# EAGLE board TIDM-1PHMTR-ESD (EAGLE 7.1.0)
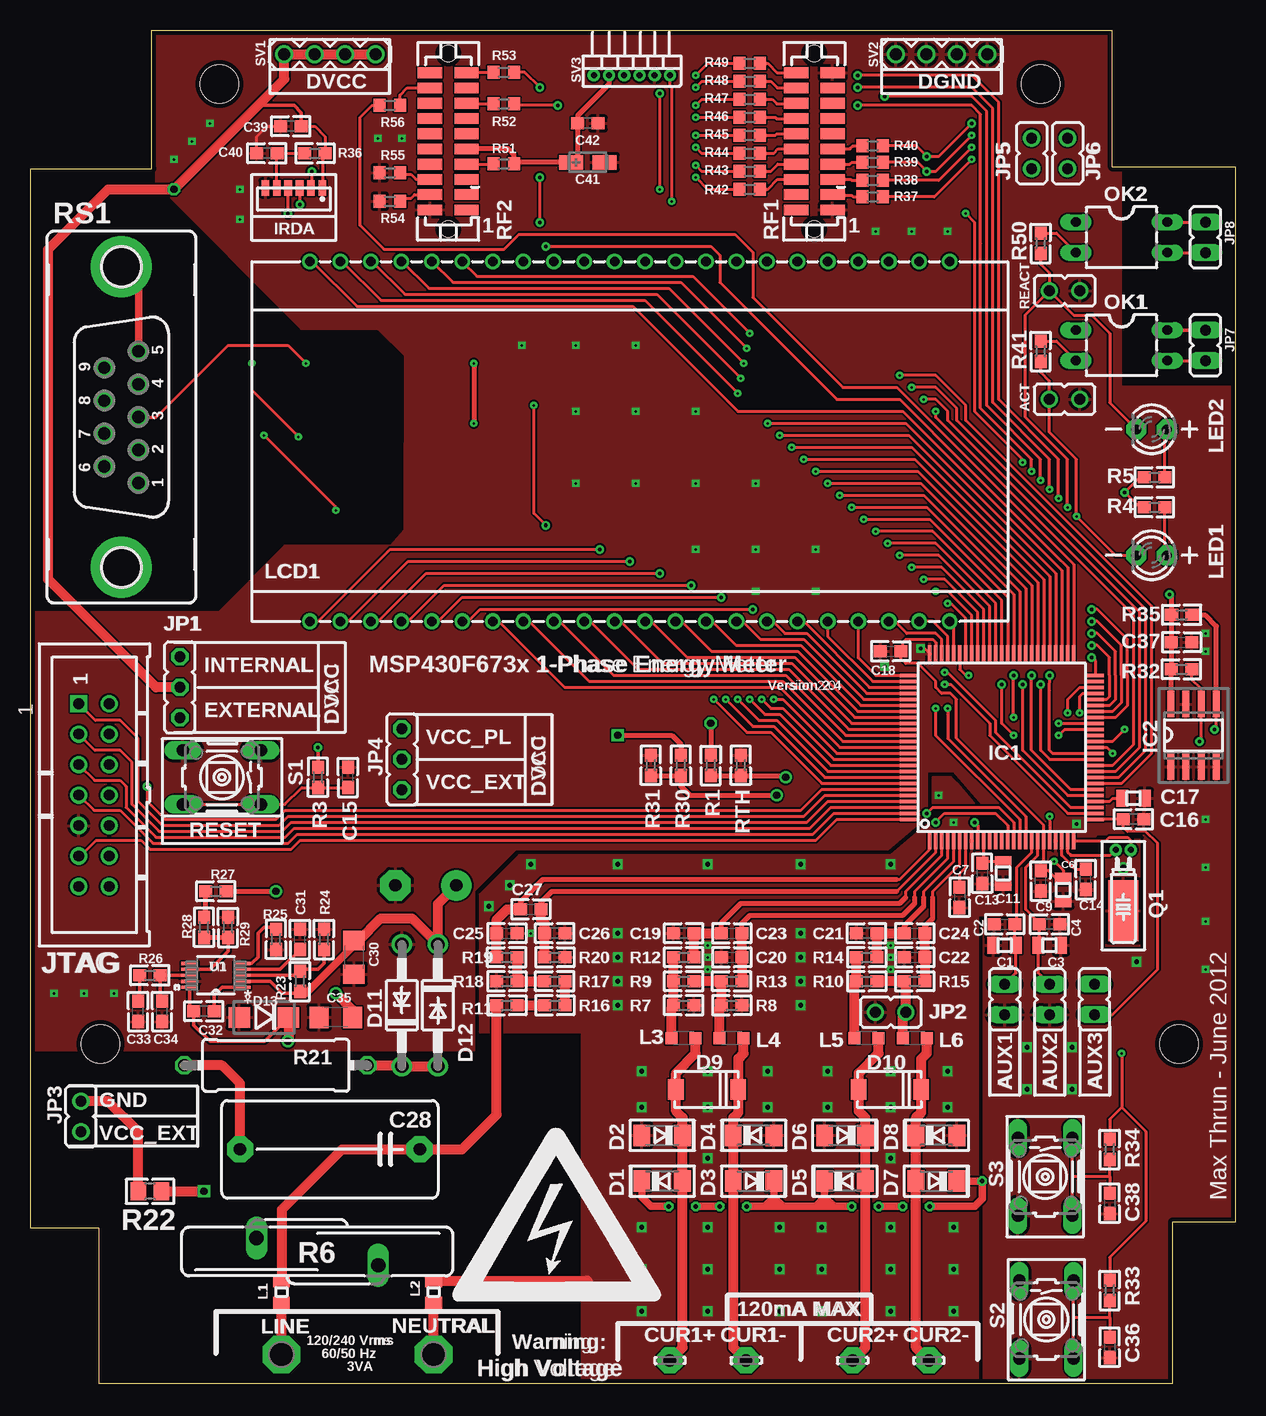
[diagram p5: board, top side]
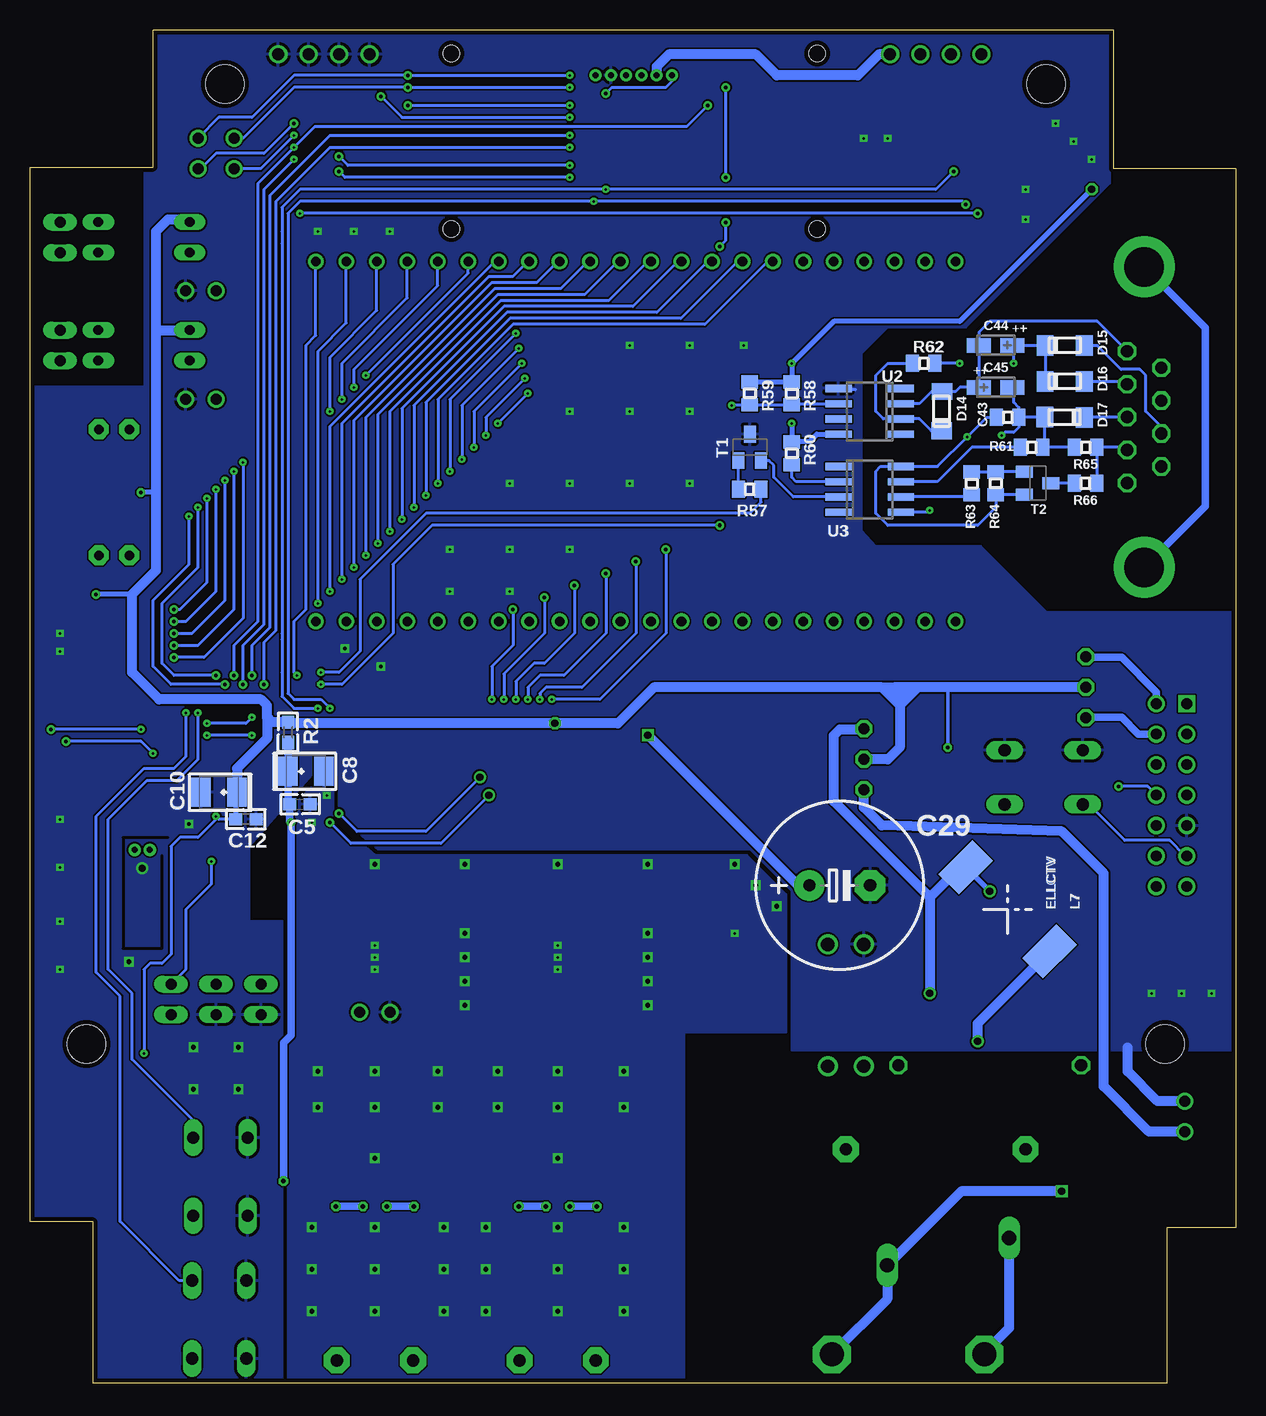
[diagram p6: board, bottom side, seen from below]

Size 100.51 x 112.78 mm. Coordinates in mm from the lower left corner, seen from the top.
Outline: 95.25,0 95.25,13.46 100.51,13.46 100.51,101.35 90.25,101.35 90.25,112.78 10.16,112.78 10.16,101.22 0,101.22 0,12.95 5.74,12.95 5.74,0 95.25,0
Copper layers (1*16): Top 0.0356mm / dielectric 1.5011mm / Bottom 0.0356mm
Design rules "typical_4pcb *": minimum track width 10mil, minimum drill 8mil, track to track 6mil, track to pad 6mil, pad to pad 6mil, via to via 6mil, smd to smd 6mil, copper to edge 15mil, drill to drill 8mil, minimum pad ring 10mil, minimum via ring 8mil, stop-mask expansion 4mil, vias tented up to drill 25mil, thermal gap 10mil
Holes 3.2 mm at 15.8,108.28 84.25,108.28 5.87,28.27 95.78,28.27
tRestrict: 4 lines
bRestrict: 4 lines

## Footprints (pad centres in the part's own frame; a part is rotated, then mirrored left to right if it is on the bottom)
JP1 = drill 0.914: 1 0,-1.27; 2 0,1.27
JP1' = drill 0.914 long: 1 0,-1.27; 2 0,1.27
0805 = smd 1 x 1.4: 1 -0.94,0; 2 0.94,0
C0603 = smd 1.1 x 1: 1 -0.85,0; 2 0.85,0
SMC_B = smd 1.6 x 2.4: + -1.5,0; - 1.5,0
C15B8 = drill 1.016 pad 2.159 octagon: 1 -7.493,0; 2 7.493,0
E5-13 = drill 1.016 pad 2.54: + -2.54,0 | drill 1.016 pad 2.54 octagon: - 2.54,0
C1206 = smd 1.6 x 1.8: 1 -1.4,0; 2 1.4,0
CT3216 = smd 2 x 1.2: + -1.4,0; - 1.4,0
CSMD0805 = smd 1.092 x 1.397: 1 -0.94,0; 2 0.94,0
LSP10 = drill 1.016 pad 2.159 octagon: MP 0,0
SOD80C = smd 1.4 x 1.8: A -1.7,0; C 1.7,0
DO-214 = smd 1.3 x 1.7: 1 0,0; 2 5.2,0
DO41Z10 = drill 1.118: A 5.08,0; C -5.08,0
DO41-10 = drill 1.118: A 5.08,0; C -5.08,0
DO214BA = smd 1.8 x 1.7: A 2.05,0; C -2.05,0
SOD-80 = smd 1.397 x 1.702: 1 1.397,-0.025; 2 -1.88,0
PZ100 = smd 1.4 x 0.3: 1 -7.8,6; 2 -7.8,5.5; 3 -7.8,5; 4 -7.8,4.5; 5 -7.8,4; 6 -7.8,3.5; 7 -7.8,3; 8 -7.8,2.5; 9 -7.8,2; 10 -7.8,1.5; 11 -7.8,1; 12 -7.8,0.5; 13 -7.8,0; 14 -7.8,-0.5; 15 -7.8,-1; 16 -7.8,-1.5; 17 -7.8,-2; 18 -7.8,-2.5; 19 -7.8,-3; 20 -7.8,-3.5; 21 -7.8,-4; 22 -7.8,-4.5; 23 -7.8,-5; 24 -7.8,-5.5; 25 -7.8,-6; 51 7.8,-6; 52 7.8,-5.5; 53 7.8,-5; 54 7.8,-4.5; 55 7.8,-4; 56 7.8,-3.5; 57 7.8,-3; 58 7.8,-2.5; 59 7.8,-2; 60 7.8,-1.5; 61 7.8,-1; 62 7.8,-0.5; 63 7.8,0; 64 7.8,0.5; 65 7.8,1; 66 7.8,1.5; 67 7.8,2; 68 7.8,2.5; 69 7.8,3; 70 7.8,3.5; 71 7.8,4; 72 7.8,4.5; 73 7.8,5; 74 7.8,5.5; 75 7.8,6 | smd 0.3 x 1.4: 26 -6,-7.8; 27 -5.5,-7.8; 28 -5,-7.8; 29 -4.5,-7.8; 30 -4,-7.8; 31 -3.5,-7.8; 32 -3,-7.8; 33 -2.5,-7.8; 34 -2,-7.8; 35 -1.5,-7.8; 36 -1,-7.8; 37 -0.5,-7.8; 38 0,-7.8; 39 0.5,-7.8; 40 1,-7.8; 41 1.5,-7.8; 42 2,-7.8; 43 2.5,-7.8; 44 3,-7.8; 45 3.5,-7.8; 46 4,-7.8; 47 4.5,-7.8; 48 5,-7.8; 49 5.5,-7.8; 50 6,-7.8; 76 6,7.8; 77 5.5,7.8; 78 5,7.8; 79 4.5,7.8; 80 4,7.8; 81 3.5,7.8; 82 3,7.8; 83 2.5,7.8; 84 2,7.8; 85 1.5,7.8; 86 1,7.8; 87 0.5,7.8; 88 0,7.8; 89 -0.5,7.8; 90 -1,7.8; 91 -1.5,7.8; 92 -2,7.8; 93 -2.5,7.8; 94 -3,7.8; 95 -3.5,7.8; 96 -4,7.8; 97 -4.5,7.8; 98 -5,7.8; 99 -5.5,7.8; 100 -6,7.8
SO-08 = smd 2.2 x 0.6: 1 -2.6,1.905; 2 -2.6,0.635; 3 -2.6,-0.635; 4 -2.6,-1.905; 5 2.6,-1.905; 6 2.6,-0.635; 7 2.6,0.635; 8 2.6,1.905
TFBS4711 = smd 0.64 x 1.27: P$1 0.625,0.635; P$2 1.575,0.635; P$3 2.525,0.635; P$4 3.475,0.635; P$5 4.425,0.635; P$6 5.375,0.635
JP2 = drill 0.914 octagon: 1 -2.54,0; 2 0,0; 3 2.54,0
MA07-2JTAG = drill 0.9 pad 1.422 square: 1 0,0 | drill 0.9 pad 1.422: 2 0,2.54; 3 2.54,0; 4 2.54,2.54; 5 5.08,0; 6 5.08,2.54; 7 7.62,0; 8 7.62,2.54; 9 10.16,0; 10 10.16,2.54; 11 12.7,0; 12 12.7,2.54; 13 15.24,0; 14 15.24,2.54
0805@1 = smd 1.092 x 1.397: 1 -0.94,0; 2 0.94,0
L2012C = smd 1 x 1: 1 -1,0; 2 1,0
ELLCTV = smd 2.4 x 4 rotated 45: 1 -3.5,-3.5; 2 3.5,3.5
TI_160SEG_LCD = drill 0.8: 1 4.826,0; 2 7.366,0; 3 9.906,0; 4 12.446,0; 5 14.986,0; 6 17.526,0; 7 20.066,0; 8 22.606,0; 9 25.146,0; 10 27.686,0; 11 30.226,0; 12 32.766,0; 13 35.306,0; 14 37.846,0; 15 40.386,0; 16 42.926,0; 17 45.466,0; 18 48.006,0; 19 50.546,0; 20 53.086,0; 21 55.626,0; 22 58.166,0; 23 58.166,29.972; 24 55.626,29.972; 29 42.926,29.972; 30 40.386,29.972; 31 37.846,29.972; 32 35.306,29.972; 33 32.766,29.972; 34 30.226,29.972; 35 27.686,29.972; 36 25.146,29.972; 37 22.606,29.972; 38 20.066,29.972; 39 17.526,29.972; 40 14.986,29.972; 41 12.446,29.972; 42 9.906,29.972; 43 7.366,29.972; 44 4.826,29.972; COM0 45.466,29.972; COM1 48.006,29.972; COM2 50.546,29.972; COM3 53.086,29.972
LED3MM = drill 0.8 pad 1.676 octagon: A -1.27,0; K 1.27,0
P1-20 = drill 2.007 pad 3.15 octagon: TP 0,0
DIL04 = drill 0.813 long: 1 -3.81,1.27; 2 -3.81,-1.27; 3 3.81,-1.27; 4 3.81,1.27
TC26H-1 = drill 0.5 pad 1.016: 1 -0.635,0; 2 0.635,0 | smd 2.54 x 5.08: 3 0,5.08
R0603 = smd 1.1 x 1: 1 -0.85,0; 2 0.85,0
S20K680-1 = drill 1.2 long: 1 -1.143,-5.08; 2 1.143,5.08
0414/15 = drill 1.016 octagon: 1 -7.62,0; 2 7.62,0
R0805 = smd 1.3 x 1.5: 1 -0.95,0; 2 0.95,0
R0603' = smd 1 x 1.1: 1 -0.85,0; 2 0.85,0
0805' = smd 1.092 x 1.397: 1 -0.94,0; 2 0.94,0
TFM-110-02-SM-D-A-K = smd 2.032 x 0.889: 1 -1.524,5.715; 2 1.524,5.715; 3 -1.524,4.445; 4 1.524,4.445; 5 -1.524,3.175; 6 1.524,3.175; 7 -1.524,1.905; 8 1.524,1.905; 9 -1.524,0.635; 10 1.524,0.635; 11 -1.524,-0.635; 12 1.524,-0.635; 13 -1.524,-1.905; 14 1.524,-1.905; 15 -1.524,-3.175; 16 1.524,-3.175; 17 -1.524,-4.445; 18 1.524,-4.445; 19 -1.524,-5.715; 20 1.524,-5.715 | hole 1.359: 0,7.303; 0,-7.303
F09VP = drill 1.016 octagon: 1 5.486,1.422; 2 2.743,1.422; 3 0,1.422; 4 -2.743,1.422; 5 -5.486,1.422; 6 4.115,-1.422; 7 1.372,-1.422; 8 -1.372,-1.422; 9 -4.115,-1.422 | drill 3.302 pad 5.08: G1 -12.522,0; G2 12.522,0
B3F-10XX = drill 1.016 long: 1 -3.251,2.261; 2 3.251,2.261; 3 -3.251,-2.261; 4 3.251,-2.261
MA04-1 = drill 1.016: 1 -3.81,0; 2 -1.27,0; 3 1.27,0; 4 3.81,0
MA06-1-1.27 = drill 0.5 pad 0.9: 1 0,0; 2 1.27,0; 3 2.54,0; 4 3.81,0; 5 5.08,0; 6 6.35,0
SOT23-BEC = smd 1 x 1.4: B -0.95,-1.1; C 0,1.1; E 0.95,-1.1
DGQ10_1P88X1P57 = smd 1.422 x 0.279: 1 -2.184,0.991; 2 -2.184,0.508; 3 -2.184,0; 4 -2.184,-0.508; 5 -2.184,-0.991; 6 2.184,-0.991; 7 2.184,-0.508; 8 2.184,0; 9 2.184,0.508; 10 2.184,0.991
SO08 = smd 0.6 x 2.2: 1 -1.905,-2.6; 2 -0.635,-2.6; 3 0.635,-2.6; 4 1.905,-2.6; 5 1.905,2.6; 6 0.635,2.6; 7 -0.635,2.6; 8 -1.905,2.6

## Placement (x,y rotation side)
ACT  [JP1]  86.25,82 270 top
AUX1  [JP1']  81.25,32 0 top
AUX2  [JP1']  85,32 0 top
AUX3  [JP1']  88.75,32 180 top
C1  4.7uF  [0805]  81.25,36.5 0 top
C2  0.1uF  [C0603]  81.25,38.25 0 top
C3  4.7uF  [0805]  85,36.5 180 top
C4  0.1uF  [C0603]  85,38.25 180 top
C5  0.1uF  [C0603]  78,48.25 0 bottom
C6  4.7uF  [0805]  86.12,41.12 90 top
C7  0.1uF  [C0603]  77.5,40.5 270 top
C8  4.7uF  [SMC_B]  77.5,51 0 bottom
C9  4.7uF  [C0603]  84.25,41.88 90 top
C10  4.7uF  [SMC_B]  84.75,49.25 180 bottom
C11  4.7uF  [0805]  81.12,42.5 90 top
C12  0.1uF  [C0603]  82.5,47 180 bottom
C13  0.1uF  [C0603]  79.38,42.5 270 top
C14  0.47uF  [C0603]  88,42 90 top
C15  0.01uF  [C0603]  26.5,50.5 90 top
C16  0.47uF  [C0603]  92,47 180 top
C17  4.7uF  [0805]  92,48.75 180 top
C18  0.1uF  [C0603]  71.75,61 0 top
C19  47pF  [C0603]  54.5,37.5 180 top
C20  47pF  [C0603]  58.5,35.5 0 top
C21  47pF  [C0603]  69.75,37.5 180 top
C22  47pF  [C0603]  73.75,35.5 0 top
C23  15nF  [C0603]  58.5,37.5 0 top
C24  15nF  [C0603]  73.75,37.5 0 top
C25  47pF  [C0603]  39.75,37.5 0 top
C26  47pF  [C0603]  43.75,37.5 180 top
C27  15nF  [C0603]  41.75,39.5 0 top
C28  0.22uF/305VAC  [C15B8]  25,19.5 180 top
C29  220uF/100V  [E5-13]  33,41.5 0 bottom
C30  2.2uF  [C1206]  27,35.5 270 top
C31  0.047uF  [C0603]  22.5,37 90 top
C32  0.047uF  [C0603]  14.5,31 180 top
C33  0.047uF  [C0603]  9,31 90 top
C34  0.047uF  [C0603]  11,31 90 top
C35  2.2uF  [C1206]  25.5,30.5 180 top
C36  0.1uF  [C0603]  90,3 270 top
C37  0.1uF  [C0603]  96,61.75 0 top
C38  0.1uF  [C0603]  90,15 270 top
C39  4.7uF  [C0603]  21.75,104.75 180 top
C40  0.1uF  [C0603]  19.75,102.5 180 top
C41  10uF  [CT3216]  46.5,101.75 0 top
C42  0.1uF  [C0603]  46.5,105 180 top
C43  0.1u  [CSMD0805]  19,80.5 0 bottom
C44  10u  [CT3216]  20,86.5 180 bottom
C45  10u  [CT3216]  20,83 0 bottom
CUR1+  [LSP10]  53.34,1.91 0 top
CUR1-  [LSP10]  59.69,1.91 0 top
CUR2+  [LSP10]  68.58,1.91 0 top
CUR2-  [LSP10]  74.93,1.91 0 top
D1  1N4148  [SOD80C]  52.7,16.85 180 top
D2  1N4148  [SOD80C]  52.7,20.66 0 top
D3  1N4148  [SOD80C]  60.33,16.85 0 top
D4  1N4148  [SOD80C]  60.33,20.66 180 top
D5  1N4148  [SOD80C]  67.94,16.85 180 top
D6  1N4148  [SOD80C]  67.94,20.66 0 top
D7  1N4148  [SOD80C]  75.56,16.85 0 top
D8  1N4148  [SOD80C]  75.56,20.66 180 top
D9  SMAJ5.0CA  [DO-214]  59.05,24.47 180 top
D10  SMAJ5.0CA  [DO-214]  74.3,24.47 180 top
D11  1N4728  [DO41Z10]  31,31.5 90 top
D12  1N4004  [DO41-10]  34,31.5 270 top
D13  B150  [DO214BA]  19.5,30.5 180 top
D14  LL103A  [SOD-80]  24.5,81.25 90 bottom
D15  LL103A  [SOD-80]  14,86.5 0 bottom
D16  LL103A  [SOD-80]  14,83.5 0 bottom
D17  LL103A  [SOD-80]  14.5,80.5 180 bottom
IC1  F6733---PZ100  [PZ100]  81,53 90 top
IC2  24C02CSN  [SO-08]  97,54 90 top
IRDA  TFBS4711-TT1  [TFBS4711]  25,100.25 180 top
JP1  [JP2]  12.5,58 270 top
JP2  [JP1]  71.75,30.93 90 top
JP3  [JP1]  4.25,22.25 180 top
JP4  [JP2]  31,52 90 top
JP5  [JP1]  83.5,102.5 0 top
JP6  [JP1]  86.5,102.5 0 top
JP7  [JP1']  98,86.5 180 top
JP8  [JP1']  98,95.5 180 top
JTAG  [MA07-2JTAG]  4.06,56.64 270 top
L1  EXCML20A  [0805@1]  20.97,7.62 90 top
L2  EXCML20A  [0805@1]  33.66,7.62 90 top
L3  BLM21BD121SN1D  [L2012C]  54.5,28.75 180 top
L4  BLM21BD121SN1D  [L2012C]  58.5,28.75 180 top
L5  BLM21BD121SN1D  [L2012C]  69.75,28.75 180 top
L6  BLM21BD121SN1D  [L2012C]  73.75,28.75 180 top
L7  ELLCTV  [ELLCTV]  19,39.5 90 bottom
LCD1  TI_160SEG_LCD  [TI_160SEG_LCD]  18.51,63.5 0 top
LED1  [LED3MM]  93.5,69 180 top
LED2  [LED3MM]  93.5,79.5 180 top
LINE  TPPAD1-20  [P1-20]  20.95,2.4 0 top
NEUTRAL  TPPAD1-20  [P1-20]  33.66,2.4 0 top
OK1  TIL191  [DIL04]  91,86.5 0 top
OK2  TIL191  [DIL04]  91,95.5 0 top
Q1  32.768  [TC26H-1]  91.15,44.45 180 top
R1  10K  [R0603]  56.75,51.5 90 top
R2  10 ohm  [R0603]  79,54.25 270 bottom
R3  47K  [R0603]  24,50.5 270 top
R4  100  [R0603]  93.75,73 180 top
R5  100  [R0603]  93.75,75.5 180 top
R6  S20K275  [S20K680-1]  23.95,10.98 90 top
R7  DNP  [R0603]  54.5,31.5 180 top
R8  0R  [R0603]  58.5,31.5 0 top
R9  13R  [R0603]  54.5,33.5 180 top
R10  13R  [R0603]  69.75,33.5 0 top
R11  330K  [R0603]  39.75,31.5 0 top
R12  1K  [R0603]  54.5,35.5 180 top
R13  1K  [R0603]  58.5,33.5 180 top
R14  1K  [R0603]  69.75,35.5 0 top
R15  1K  [R0603]  73.75,33.5 0 top
R16  330K  [R0603]  43.75,31.5 0 top
R17  330K  [R0603]  43.75,33.5 180 top
R18  3K  [R0603]  39.75,33.5 0 top
R19  100  [R0603]  39.75,35.5 180 top
R20  1K  [R0603]  43.75,35.5 0 top
R21  560R/3W  [0414/15]  20.5,26.5 0 top
R22  0  [R0805]  10,16 180 top
R23  1.8M  [R0603]  22.5,33.5 90 top
R24  59k  [R0603]  24.5,37 90 top
R25  332k  [R0603]  20.5,37 270 top
R26  332k  [R0603]  10,34 180 top
R27  51  [R0603]  15.5,41 180 top
R28  316k  [R0603]  14.5,38 270 top
R29  100k  [R0603]  16.5,38 90 top
R30  5K  [R0603]  54.25,51.5 270 top
R31  5K  [R0603]  51.75,51.5 270 top
R32  10K  [R0603]  96,59.5 180 top
R33  100k  [R0603]  90,7.75 90 top
R34  100k  [R0603]  90,19.5 90 top
R35  10K  [R0603]  96.02,64.04 180 top
R36  47  [R0603]  23.75,102.5 0 top
R37  0  [R0603']  70.25,98.88 180 top
R38  0  [R0603']  70.25,100.25 180 top
R39  0  [R0603']  70.25,101.75 180 top
R40  0  [R0603']  70.25,103.12 180 top
R41  1K  [R0603]  84.25,86 90 top
R42  0  [R0603']  60,99.5 180 top
R43  0  [R0603']  60,101 180 top
R44  0  [R0603']  60,102.5 180 top
R45  0  [R0603']  60,104 180 top
R46  0  [R0603']  60,105.5 180 top
R47  0  [R0603']  60,107 180 top
R48  0  [R0603']  60,108.5 180 top
R49  0  [R0603']  60,110 180 top
R50  1K  [R0603]  84.25,95 90 top
R51  0  [R0603']  39.5,101.63 180 top
R52  0  [R0603']  39.5,106.63 180 top
R53  0  [R0603']  39.5,109.25 180 top
R54  0  [R0603']  30,98.5 180 top
R55  0  [R0603']  30,100.88 180 top
R56  0  [R0603']  30,106.5 180 top
R57  2.2k  [0805']  40.5,74.5 180 bottom
R58  -  [0805']  37,82.5 90 bottom
R59  2.2k  [0805']  40.5,82.5 270 bottom
R60  68  [0805']  37,77.5 270 bottom
R61  DNP  [0805']  17,78 0 bottom
R62  1k  [0805']  26,85 0 bottom
R63  1k  [0805']  22,75 90 bottom
R64  10k  [0805']  20,75 270 bottom
R65  1.5k  [0805']  12.5,78 0 bottom
R66  220  [0805']  12.5,75 180 bottom
REACT  [JP1]  86.27,91.03 270 top
RF1  [TFM-110-02-SM-D-A-K]  65.39,103.5 180 top
RF2  [TFM-110-02-SM-D-A-K]  34.87,103.5 180 top
RS1  [F09VP]  7.62,80.52 270 top
RTH  10K Thermistor  [R0603]  59.25,51.5 270 top
S1  [B3F-10XX]  16,50.5 180 top
S2  [B3F-10XX]  84.73,5.32 270 top
S3  [B3F-10XX]  84.63,17.22 270 top
SV1  [MA04-1]  25,110.75 0 top
SV2  [MA04-1]  76,110.75 0 top
SV3  [MA06-1-1.27]  47,109 0 top
T1  BC860B/BC857B  [SOT23-BEC]  40.5,78 0 bottom
T2  BC860B/BC857B  [SOT23-BEC]  16.5,75 270 bottom
U1  TPS5401_DGQ_10  [DGQ10_1P88X1P57]  15.5,34 180 top
U2  PS8802  [SO08]  30.5,81 90 bottom
U3  PS8802  [SO08]  30.5,74.5 270 bottom

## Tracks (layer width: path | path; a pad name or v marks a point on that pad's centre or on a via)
+9V  (via drill 0.6)
  Top 0.305: U1.2 20.01,33.49 21,32.5 22.35,32.5 R23.1
  Top 0.406: R30.1 54.25,53.25 53.5,54 v49,54
  Top 0.61: 27.4,36.9 C30.1 27,36.5 23,32.5 22.65,32.5 R23.1
  Top 0.813: 27.4,36.9 29.25,38.75 31.83,38.75 D12.C 34,39.96 C29.+
  Bottom 0.813: C29.+ 36.5,41.5 v49,54
+12V  (via drill 0.2)
  Top 0.254: v18.5,85 18.5,82.75 v22.38,78.88
  Bottom 0.254: D16.2 D15.2 18.5,86.5 | T2.E R64.2 20,73 21.5,71.5 29,71.5 30,72.5 30,76 29.59,76.41 U3.8 24.84,76.41 v22.38,78.88 20.75,80.5 C43.1 | 18.5,86.5 C44.+ | v18.5,85 18.5,86.5
+12V2
  Bottom 0.254: D15.1 11.53,86.47 9.55,84.5 8,84.5 7.5,84 7.5,81 6.2,79.7 RS1.7
+12V3
  Bottom 0.254: D16.1 9.26,83.47 RS1.4
-12V  (via drill 0.2)
  Top 0.254: v19.5,79 25.5,73 v25.5,72.75
  Bottom 0.254: R65.1 R61.2 15.9,78.16 D17.1 18.04,80.53 C43.2 | C43.2 18.06,81.31 18.5,81.75 18.5,82.9 C45.- | C43.2 18.06,79.69 18.5,79.25 19.25,79.25 v19.5,79 | U3.5 25.66,72.59 v25.5,72.75
ACT  (via drill 0.2, 0.3)
  Top 0.254: IC1.36 85,52 84.25,52.75 v84.25,58.25 | R41.1 84.25,84.25 84.98,83.52 ACT.1 84.98,79.27 87.25,77 v87.25,72.25 90.5,69 LED1.K
  Bottom 0.254: v84.25,58.25 88.75,58.25 90.25,59.75 90.25,65.25 87.25,68.25 v87.25,72.25
AGND  (via drill 0.2, 0.4)
  Top 0.813: L2.2 46.44,8.56 46.5,8.5
  other vias: 51,13 51,9.5 51,6 56.5,13 56.5,9.5 56.5,6 62.5,13 62.5,9.5 62.5,6 66,6 66,9.5 66,13 71.75,13 71.75,9.5 71.75,6 77,13 77,9.5 77,6 76.5,26 76.5,23 66.5,23 66.5,26 61.5,26 61.5,23 51,23 51,26 49,31.5 49,33.5 49,35.5 49,37.5 64.25,37.5 64.25,35.5 64.25,33.5 64.25,31.5 71.75,43.25 64.25,43.25 56.5,43.25 49,43.25 41.75,43.25 40,41.5 38.25,39.75 71.75,36.5 71.75,35.5 71.75,34.5 56.5,36.5 56.5,35.5 56.5,34.5 41.75,37.5 77,46.75 75.75,49 56.5,23 56.5,26 56.5,18.75 71.75,18.75 71.75,23 71.75,26
  pour Bottom: 81.75,44.5 81.75,39 79,39 79,-0.5 46,-0.5 46,29.25 37.5,29.25 37.5,40.75 40.75,44 71.75,44 75,46.75 75.25,47 75.25,50 76.75,50 80,46.75
  pour Top: 81.75,44.5 81.75,39 79,39 79,-1.5 46,-1.5 46,29.25 37.5,29.25 37.5,40.75 40.75,44 71.75,44 75,46.75 75.25,47 75.25,50.5 76.75,50.5 77.25,50 80,46.75
AUXVCC1
  Top 0.254: C4.2 84.29,38.35 | C4.2 83.86,38.35 | C4.2 84.15,38.35 83,39.5 83,43 84,44 IC1.19 | C4.2 84.15,36.59 C3.2 84.06,34.21 AUX2.2
AUXVCC2
  Top 0.254: 82.09,36.74 82.26,36.58 C1.2 | IC1.18 83.5,44.25 82.25,43 82.25,38.4 C2.2 82.1,36.59 C1.2 | C1.2 82.19,34.21 AUX1.2
AVCC  (via drill 0.3, 0.38)
  Top 0.254: IC1.9 79,46.5 v78.75,46.75
  Top 0.61: D7.C v79.38,16.85 79.38,15.38 78.75,14.75 v75,14.75 | D1.C 51.01,15.49 51.75,14.75 v53.25,14.75 | v55.5,14.75 v57.5,14.75 | v59.75,14.75 61.25,14.75 | 61.25,14.75 62,14.75 | 62,14.75 62.75,14.75 | 62.75,14.75 65.5,14.75 | 65.5,14.75 66.25,14.75 | 66.25,14.75 67,14.75 | 67,14.75 v68.5,14.75 | D3.C 62.02,14.78 62,14.75 | D3.C 62.02,15.53 61.25,14.75 | D3.C 62.02,15.47 62.75,14.75 | D5.C 66.25,14.76 66.25,14.75 | D5.C 66.25,15.49 65.5,14.75 | D5.C 66.25,15.51 67,14.75 | v70.75,14.75 v72.75,14.75
  Bottom 0.406: C5.1 79,48.65 | v78.75,46.75 78.85,46.85
  Bottom 0.61: R2.2 C8.+ 79,48.65 | 78.85,46.85 C5.1 | v79.38,16.85 79.38,28.38 78.75,29 v78.75,46.75 | v78.75,46.75 | v53.25,14.75 v55.5,14.75 | v57.5,14.75 v59.75,14.75 | v68.5,14.75 v70.75,14.75 | v72.75,14.75 v75,14.75
BT1  (via drill 0.2)
  Top 0.254: v86.5,55.88 86.5,57 87.5,58 IC1.48 | S3.2 86.89,17.25 | 86.89,17.25 S3.1 | 90,17.25 C38.1 | 90,17.25 R34.1 | 86.89,17.25 90,17.25
  Bottom 0.254: S3.1 86.89,20.55 86.87,20.57 86.87,21.87 92,27 92,32.5 94,34.5 94,47 90.75,50.25 88.25,50.25 86.5,52 v86.5,55.88
BT2  (via drill 0.2)
  Top 0.254: v87.5,55.88 87.5,57.25 87.75,57.5 IC1.47 | 90,5.5 C36.1 | 90,5.5 R33.1 | S2.2 87,5.5 | 87,5.5 S2.1 | 87,5.5 90,5.5
  Top 0.406: C36.1 89.92,4.06
  Bottom 0.254: S2.1 88.07,8.57 93,13.5 93,32.25 95,34.25 95,47.25 91,51.25 88.5,51.25 87.5,52.25 v87.5,55.88
COM0  (via drill 0.2)
  Top 0.254: v72.5,84 75.5,84 78,81.5 78,80.25 93.5,64.75 93.5,52.5 91,50 IC1.32
  Bottom 0.254: LCD1.COM0 63.98,92.52 v72.5,84
COM1  (via drill 0.2)
  Top 0.254: v73.5,83 75.5,83 77.25,81.25 77.25,80.25 93,64.5 93,52.75 90.75,50.5 IC1.33
  Bottom 0.254: LCD1.COM1 66.52,91.48 73.5,84.5 v73.5,83
COM2  (via drill 0.2)
  Top 0.254: v74.5,82 75.5,82 76.5,81 76.5,80.25 92.5,64.25 92.5,53 90.5,51 IC1.34
  Bottom 0.254: LCD1.COM2 69.06,90.44 74.5,85 v74.5,82
COM3  (via drill 0.2)
  Top 0.254: v75.5,81 75.5,80.5 92,64 92,53.25 90.25,51.5 IC1.35
  Bottom 0.254: LCD1.COM3 71.6,89.4 75.5,85.5 v75.5,81
DGND  (via drill 0.2, 0.3, 0.4, 0.6)
  Top 0.254: IC2.1 95.11,51.19 95.23,51.06 95.15,50.97 | IC2.2 96.44,51.26 96.5,51.32 | IC2.7 96.44,56.46 96.5,56.4 96.38,56.27 | IC2.3 97.58,51.26 97.52,51.32 97.46,51.26 | C1.1 80.22,36.58 | C4.1 85.81,38.35 85.99,38.53 | C3.1 85.74,36.14 | C14.1 88.1,40.89 | v74.25,61.25 74.55,61.25 IC1.75 | C40.2 18.9,103.9 19.75,104.75 C39.2
  Top 0.813: JP3.1 6.48,23.52 9,21 9,16.05 R22.2
  Bottom 0.254: 31.68,82.81 U2.5 31.67,82.8
  Bottom 0.813: 9,28 9,26 6.52,23.52 JP3.1
  other vias: 91.15,42.93 71.25,59.75 83.12,24.5 83.12,28 86.88,28 86.88,24.5 87.25,46.62 98,62.5 98,61 45.5,75 45.5,86.5 45.5,81 50.5,86.5 50.5,81 50.5,75 55.5,75 55.5,81 60.5,75 2,32.5 4.5,32.5 7,32.5 92.25,35.12 60.5,69.5 55.5,69.5 60.5,66 65.5,66 65.5,69.5 41,86.5 70.5,96 76.5,96 73.5,96 31,103.75 12,102 15,105 13.5,103.5 17.5,99.5 17.5,97 29,103.75 98,47 98,34.5 98,38.5 98,43
  pour Top: -0.55,27.71 -0.55,64.26 15.75,64.26 21.25,69.79 30.09,69.79 31.22,71.07 31.28,85.63 29.01,87.84 29.01,87.88 22.61,87.88 10.5,100 10.5,113.5 89.92,113.52 89.92,101.09 90.93,101.09 90.93,83.06 103.83,83.06 103.83,12.22 96.74,12.22 96.75,-1.5 79.5,-1.5 79.5,38.5 82.25,38.5 82.25,44.75 80.25,47.25 77,51 74.75,51 74.75,47.25 71.5,44.5 40.5,44.5 37,41 37,27.75
  pour Bottom: -0.53,27.71 -0.53,64.26 15.75,64.26 21.25,69.75 30,69.75 31.21,71.1 31.21,85.79 29,88 22.5,88 10.5,100 10.5,114 89.92,114.02 89.92,101.09 90.93,101.09 90.93,83.06 101.83,83.06 101.83,12.97 95.74,12.97 95.75,-0.5 79.5,-0.5 79.5,38.5 82.25,38.5 82.25,44.75 77,50.75 74.75,50.75 74.75,47.25 71.5,44.5 40.5,44.5 37,41 37,27.75
  pour Top: 86.32,46.74 91.15,46.74 91.65,45.97 92.67,45.72 92.67,36.32 89.62,36.32 89.62,43.69 87.08,43.69 86.07,44.7 86.07,46.48
DVCC  (via drill 0.2, 0.3, 0.6)
  Top 0.254: C39.1 23.75,104.75 24.6,103.9 R36.2 24.38,102.28 IRDA.P$1 | R5.2 92.5,75.5 v91.25,74.25 92.5,73 R4.2 | R33.2 90,10.5 93,13.5 93,21 91,23 | IC1.21 85,46.5 v85,47.25 | 91,23 90,22 R34.2 | v91,27.5 91,23
  Top 0.305: v24,53 R3.1 | C39.1 22.6,105.9 22,106.5 19,106.5
  Top 0.406: IC2.8 95.09,59.45 R32.2 C37.1 95.15,64.02 | 95.15,64.02 R35.2 | 95.15,64.02 95.15,65.6 v95,65.75 | SV3.2 48.27,108.27 45.65,105.65 C42.2 45.65,102.3 C41.+ 40.48,101.75 R51.1 40.35,102.4 39.88,102.86 RF2.9 | v37,85 v37,80 | v56.75,55 R1.2
  Top 0.813: JP1.2 10.5,58 1.5,67 1.5,94.5 6.5,99.5 v12,99.5 19,106.5 21.19,108.69 SV1.1 SV1.2 SV1.3 SV1.4
  Bottom 0.254: v91.25,74.25 | v91,27.5 91,34.5 90.5,35 89.5,35 88.75,35.75 88.75,44.75 88,45.5 86.5,45.5 85,47 v85,47.25 84.75,47 C12.2 | R60.1 36.94,78.5 | v95,65.75
  Bottom 0.305: 24,58 v24,53
  Bottom 0.406: 83.35,49.21 C12.2 | 92,65.75 v95,65.75 | 90,74.25 v91.25,74.25 | v12,99.5 23,88.5 33.5,88.5 v37,85 R58.2 R59.1 | v37,80 R60.1 | U2.8 34.91,79.09 35.5,78.5 36.94,78.5
  Bottom 0.813: 90,87.5 90,74.25 90,67.75 92,65.75 92,59.25 89.75,57 81.25,57 80.75,56.5 80.75,55.5 | 90,87.5 90,96 89,97 87.13,97 OK2.1 | OK1.1 90,87.75 90,87.5 | 83.35,49.21 C10.+ 83.25,51.25 80.75,53.75 80.75,55.5 | JP1.2 24,58 26.5,58 | 26.5,58 27.5,58 | 27.5,58 28,58 | 29.5,58 28.5,58 | 28,58 28.5,58 | 29.5,58 48.5,58 51.5,55 v56.75,55 78.9,55 R2.1 80.35,55.1 80.75,55.5 | SV1.4 29.75,110.75 31.5,109 38.25,109 40,110.75 47.25,110.75 48.27,109.73 SV3.2 | JP4.2 29,52 28,53 28,56.5 | 28,57.5 28,58 | 28,56.5 29.5,58 | 26.5,58 28,56.5 | 27.5,58 28,57.5 | 28,56.5 28,57.5 | 28,57.5 28.5,58
EXT_VCC
  Bottom 0.813: JP3.2 7.23,20.98 11,24.75 11,42.5 14.5,46 29.5,46.5 31,48 JP4.1
GND1
  Top 0.61: RS1.5 9.04,91.62 RS1.G1
  Bottom 0.254: U2.3 26.36,81.64 25.35,82.65 D14.1 23.35,82.65 23,83 C45.+ C44.- 21.4,87.6 20.5,88.5 11.54,88.5 RS1.5
  Bottom 0.61: RS1.G2 2.54,73.08 2.54,87.96 RS1.G1
I1+
  Top 0.254: IC1.3 76,44 73,41 73,40.5
  Top 0.406: C23.1 57.65,38.4 59.25,40 72.5,40 73,40.5
  Top 0.813: R12.1 C19.1 | C19.1 | C19.1 C23.1
I1-
  Top 0.254: IC1.4 76.5,43.75 73.75,41 73.75,40.5
  Top 0.406: C23.2 59.35,38.35 60,39 72.75,39 73.75,40 73.75,40.5
  Top 0.813: C20.2 R13.1 | C20.2 | C20.2 C23.2 | C23.2
IN+
  Top 0.254: IC1.5 77,43.5 74.5,41 74.5,40.5
  Top 0.406: C24.1 72.9,38.15 74.5,39.75 74.5,40.5
  Top 0.813: C24.1 C21.1 R14.2 | C24.1
IN-
  Top 0.254: IC1.6 77.5,43.25 75.25,41 75.25,40.5
  Top 0.406: C24.2 74.6,38.1 75.25,38.75 75.25,40.5
  Top 0.813: C22.2 C24.2 | C22.2 | C22.2 R15.2 | C22.2
IR_SD  (via drill 0.2, 0.3)
  Top 0.254: IC1.50 88.8,60.2 v88.5,60.5 | v82.75,76.75 82.75,77 78.75,81 78.75,95 | 78.75,95 | 78.75,95 78.75,96.75 v78,97.5 | v21.5,97.5 21.5,99.59 IRDA.P$4
  Bottom 0.254: v88.5,60.5 86,60.5 82.75,63.75 v82.75,76.75 | v21.5,97.5 v78,97.5
JTAG_EXT
  Bottom 0.61: JTAG.4 8.1,54.1 9.5,55.5 12.46,55.5 JP1.3
JTAG_INT
  Bottom 0.61: JTAG.2 6.6,57.6 9.5,60.5 12.46,60.5 JP1.1
LCDCAP
  Top 0.254: IC1.29 90,48.5 90.25,48.75 C17.2 | C17.2
LINE-VA
  Top 0.813: L1.2 21,8.59 21,14.5 26,19.5 C28.1 36,19.5 38.9,22.4 R11.1
N$1
  Top 0.813: R21.1 16,26.5 17.5,25 C28.2
N$2
  Top 0.254: IRDA.P$5 20.57,102.47 C40.1 R36.1
N$3
  Top 0.813: R21.2 30.42,26.5 D11.C D12.A
N$5
  Top 0.813: L1.1 20.97,2.42 LINE.TP
  Bottom 0.813: R6.2 18.88,4.62 20.95,2.54 LINE.TP
N$7
  Top 0.305: U1.3 22.15,34 R23.2 22.65,34.5 24,34.5 24.5,35 R24.1
N$12
  Top 0.305: U1.4 20.49,34.51 20.5,34.5 20.85,34.5 C31.1
N$13
  Top 0.305: U1.5 18.49,34.99 19,35.5 19,37.5 19.5,38 20.35,38 R25.1
N$14
  Bottom 0.254: D14.2 25.37,79.37 26.36,80.36 U2.2 29.36,80.36 30,81 30,84 29,85 R62.1
N$15
  Bottom 0.254: U3.7 24.86,75.14 22,78 R61.1
N$16
  Bottom 0.254: U3.6 22.2,73.86 R63.1
N$17
  Bottom 0.254: R66.2 T2.C
N$18
  Bottom 0.254: R57.2 T1.B
N$19
  Top 0.813: CUR1+.MP 54.41,2.97 D1.A D2.C 54.41,22.14 53.85,22.68 D9.2 53.85,25.86 55.5,27.5 L3.1
N$20
  Top 0.813: CUR1-.MP 58.62,2.97 D3.A D4.C 58.62,22.14 59.05,22.57 D9.1 59.05,27.05 59.5,27.5 L4.1
N$21
  Top 0.813: CUR2+.MP 69.64,2.97 D5.A D6.C 69.64,22.14 69.09,22.68 D10.2 69.09,25.84 70.75,27.5 L5.1
N$22
  Top 0.813: CUR2-.MP 73.86,2.97 D7.A D8.C 73.86,22.14 74.3,22.57 D10.1 74.3,27.05 74.75,27.5 L6.1
N$23
  Top 0.305: R26.2 9.15,32.5 C33.2
N$24
  Top 0.813: R15.1 R10.2 | R15.1 | L6.2 72.75,30.66 JP2.1 73.03,33.38 R15.1
N$25
  Top 0.406: R28.1 14.65,39 R27.2
N$26
  Top 0.305: U1.8 R26.1 10.85,32.5 C34.2
N$27
  Top 0.813: L4.2 57.5,31.35 R8.1 | R9.1 R13.2 R8.1 | R8.1
N$28
  Top 0.305: C32.1 15.35,32.35 16,33 U1.1
N$29  (via drill 0.6)
  Top 0.305: U1.10 13.32,31.33 C32.2 13.65,29.85 15,28.5 19.55,28.5 D13.C
  Top 0.813: v21.5,28.5 21.55,28.55 D13.C
  Bottom 0.813: L7.1 21.5,30 v21.5,28.5
N$30
  Bottom 0.254: T2.B R64.1 R63.2
N$31
  Top 0.813: R14.1 R10.1 68.75,33.35 L5.2
N$32
  Top 0.813: R17.2 R18.2 R19.1
N$34
  Top 0.305: U1.7 15.01,34.51 16.5,36 R29.1
  Top 0.406: R29.1 R28.2
N$35
  Top 0.254: R37.2 68.62,98.88 68.5,99 66.97,99 RF1.3
N$38
  Top 0.254: C16.2 IC1.26 | C16.2 | C16.2 91.15,46.35 91.5,46 93,46 94,45 94,34.5 90.23,30.73 AUX3.2
N$39
  Top 0.813: R11.2 R16.1
N$42
  Top 0.813: L3.2 53.5,31.35 R7.2 R9.2 R12.2 | R12.2
N$45
  Top 0.254: RF1.5 68.42,100.33 68.5,100.25 R38.2
N$49
  Bottom 0.254: U3.2 36.63,75.14 37,75.5 R60.2
N$50
  Top 0.254: RF2.7 38.62,101.59 R51.2
N$51
  Top 0.254: RF2.4 32.05,99.06 31.75,98.75 31.1,98.75 R54.1
N$52
  Top 0.254: R52.2 36.44,106.62 RF2.15
N$53
  Top 0.254: RF2.6 32.17,100.33 31.75,100.75 30.98,100.75 R55.1
N$55
  Top 0.254: R44.1 62,102.5 62.37,102.86 RF1.10
N$56
  Top 0.254: R45.1 62.12,104 62.25,104.12 63.86,104.12 RF1.12
N$57
  Top 0.254: R46.1 62.12,105.5 62.25,105.38 63.84,105.38 RF1.14
N$59
  Top 0.254: R47.1 61.88,107 62.25,106.62 63.82,106.62 RF1.16
N$60
  Top 0.254: R48.1 61.75,108.5 62.3,107.94 RF1.18
N$61
  Top 0.254: R49.1 61.5,110 62.28,109.22 RF1.20
N$81
  Top 0.254: R53.2 36.43,109.25 RF2.19
N$83
  Top 0.254: RF2.18 31.45,107.94 30.85,107.35 R56.1
N$85
  Top 0.254: RF1.7 68.34,101.59 68.5,101.75 R39.2
N$86
  Top 0.254: R40.2 68.62,103.12 68.36,102.86 RF1.9
N$87
  Top 0.254: R43.1 61.75,101 62.34,101.59 RF1.8
N$88
  Top 0.254: 63.82,100.38 RF1.6 62.33,100.33 61.5,99.5 R42.1
N$104
  Top 0.254: R4.1 94.6,69.17 LED1.A
N$105
  Top 0.254: R5.1 94.6,79.33 LED2.A
N$109
  Top 0.305: OK1.4 JP7.1
N$113
  Top 0.254: R50.2 85.57,95.85 OK2.2
N$114
  Top 0.254: R41.2 85.57,86.85 OK1.2
N$117
  Top 0.254: OK1.3 JP7.2
N$118
  Top 0.254: OK2.4 JP8.1
N$119
  Top 0.254: OK2.3 JP8.2
N$455
  Bottom 0.254: U3.3 36.87,73.86 38.5,75.5 38.5,76.5 38.9,76.9 T1.E
NEUTRAL  (via drill 0.6)
  Top 0.813: NEUTRAL.TP L2.1 | R22.1 v14.5,16
  Bottom 0.813: NEUTRAL.TP 29.04,7.03 R6.1 22.87,16 v14.5,16
PL_VCC  (via drill 0.6)
  Top 0.406: R27.1 v20.5,41
  Top 0.813: v25.5,32.5 26.9,31.1 C35.1
  Bottom 0.406: v20.5,41 L7.2
  Bottom 0.61: 31.04,54.5 JP4.3
  Bottom 0.813: 25.5,40.5 v25.5,32.5 | 25.5,40.5 33.5,48.5 33.5,54 33,54.5 31.04,54.5 | L7.2 23,43 25.5,40.5
REACT  (via drill 0.2, 0.3)
  Top 0.254: IC1.37 85.25,52.5 85,52.75 85,57.72 v85,59 | v86.5,73 86.5,77 83,80.5 83,89.04 REACT.1 87.03,89 88.5,89 90,87.5 90,81.73 LED2.K | REACT.1 85,92.5 84.25,93.25 R50.1
  Top 0.305: REACT.1
  Bottom 0.254: v85,59 88.5,59 89.5,60 89.5,65 86.5,68 v86.5,73
RESET
  Top 0.254: JTAG.11 4.19,43.94 5.5,45.25 9.25,45.25 10,44.5 21.75,44.5 22.5,45.25 65.5,45.25 67.25,47 IC1.100 | C15.1 R3.2 22.65,49.65 21.24,48.24 S1.1 S1.2
  Bottom 0.254: JTAG.11 4.19,43.94 5.5,45.25 9.25,45.25 12.25,48.25 12.74,48.25 S1.2
RF_CCA  (via drill 0.2, 0.3)
  Top 0.254: IC1.41 86.25,54.5 v85.75,54 | v82,54 81,55 81,57.5 v81,58.25 | R44.2 56,102.5 v55.5,103
  Bottom 0.254: v82,54 v85.75,54 | v81,58.25 81,59.5 | 81,59.5 | 81,59.5 81,61.75 80,62.75 80,98.5 75.5,103 v55.5,103
RF_CLK  (via drill 0.2, 0.3)
  Top 0.254: IC1.46 89.75,57 90,57.25 90,59 | 90,59 | 90,59 90,60.5 89,61.5 v88.5,61.5 | v83.5,76 83.5,77 79.25,81.25 79.25,95 | 79.25,95 | 79.25,95 79.25,105.75 78.5,106.5 v69,106.5 | R47.2 56,107 v55.5,106.5
  Bottom 0.254: v88.5,61.5 86.5,61.5 83.5,64.5 v83.5,76 | v69,106.5 v55.5,106.5
RF_CS  (via drill 0.2, 0.3)
  Top 0.254: IC1.45 90,56.5 90.5,57 90.5,59 | 90.5,59 | 90.5,59 90.5,61 89,62.5 v88.5,62.5 | v84.25,75.25 84.25,77 79.75,81.5 79.75,106 78.5,107.25 v71.25,107.25 | v55.5,105.5 R46.2 | v55.5,105.5
  Bottom 0.254: v88.5,62.5 87,62.5 84.25,65.25 v84.25,75.25 | v71.25,107.25 69.5,105.5 v55.5,105.5
RF_FIFO  (via drill 0.2, 0.3)
  Top 0.254: R42.2 56.5,99.5 v55.5,100.5 | v78.5,104 75.5,101 v74.75,101 74,101.75 R39.1
  Bottom 0.254: v55.5,100.5 74.25,100.5 v74.75,101 | JP5.1 81.27,101.23 v78.5,104
RF_FIFOP  (via drill 0.2, 0.3)
  Top 0.254: R43.2 56,101 v55.5,101.5 | v78.5,105 75.75,102.25 v74.75,102.25 73.88,103.12 R40.1
  Bottom 0.254: v55.5,101.5 74,101.5 v74.75,102.25 | JP6.1 86.27,101.23 85,102.5 81,102.5 v78.5,105
RF_GPIO1  (via drill 0.3)
  Top 0.254: IC1.52 86.5,68 85.5,69 | 85.5,69 | 78,76.5 85.5,69 | 78,76.5 | 78,76.5 72.5,82 67.25,82 57.5,91.75 57.5,94 56.75,94.75 v43,94.75 | R53.1 41.25,109.25 v42.5,108 | v42.5,96.75 v42.5,100.5
  Bottom 0.254: v43,94.75 42.5,95.25 v42.5,96.75 | v42.5,100.5 v42.5,108
RF_GPIO2
  Top 0.254: IC1.51 87,68.25 72.25,83 67.75,83 60.25,90.5 60.25,94.25 58.75,95.75 40.75,95.75 39.5,94.5 29.5,94.5 27.5,96.5 27.5,105.5 28.5,106.5 R56.2 | R56.2
RF_RESETCC  (via drill 0.2, 0.3)
  Top 0.254: IC1.31 86.75,49.5 83.5,52.75 v83.5,59 | v44,106.5 40.48,106.5 R52.1 | R38.1 75.75,100.25 v78.5,103
  Bottom 0.254: v83.5,59 83.5,61.5 81.5,63.5 81.5,100 v78.5,103 76.75,104.75 45.75,104.75 v44,106.5
RF_SFD  (via drill 0.2, 0.3)
  Top 0.254: v85.75,55 IC1.42 | v82,55.5 v82,59 | v55.5,104 R45.2 | v55.5,104
  Bottom 0.254: v85.75,55 82.5,55 v82,55.5 | v82,59 82,59.5 82,61.5 80.5,63 80.5,99 75.5,104 v55.5,104
RF_SIMO  (via drill 0.2, 0.3)
  Top 0.254: IC1.44 90.25,56 91,56.75 91,59 | 91,59 | 91,59 91,61.5 89,63.5 v88.5,63.5 | v85,74.5 85,77 80.25,81.75 80.25,106.25 78.5,108 v69,108 | R48.2 56,108.5 v55.5,108
  Bottom 0.254: v88.5,63.5 87.5,63.5 85,66 v85,74.5 | v55.5,108 v69,108 78.5,108 82.73,103.77 JP5.2
RF_SOMI  (via drill 0.2, 0.3)
  Top 0.254: IC1.43 90.5,55.5 91.5,56.5 91.5,59 | 91.5,59 | 91.5,59 91.5,62 89,64.5 v88.5,64.5 | v85.75,73.75 85.75,77 80.75,82 80.75,106.75 78.5,109 v69,109 | R49.2 56.5,110 v55.5,109
  Bottom 0.254: v88.5,64.5 88,64.5 85.75,66.75 v85.75,73.75 | v55.5,109 v69,109 78.5,109 82,105.5 84.77,105.5 JP6.2
RF_VREG_EN  (via drill 0.2, 0.3)
  Top 0.254: IC1.30 86.5,49 82.75,52.75 v82.75,58.25 | R37.1 75.38,98.88 v78.5,102
  Bottom 0.254: v82.75,58.25 82.75,61.5 81,63.25 81,99.5 v78.5,102
RS232_RXD  (via drill 0.2, 0.3)
  Top 0.254: v76.25,58.25 76.75,58.25 80,55 80,54 86.5,47.5 IC1.27 | v42,81.5 42,72.5 v43,71.5
  Bottom 0.254: v43,71.5 67,71.5 70.25,68.25 70.25,62.5 74.5,58.25 v76.25,58.25 | U2.6 36.92,81.64 R58.1 R59.2 41.94,81.56 v42,81.5
RS232_TXD  (via drill 0.2)
  Top 0.254: v76.25,59.25 76.5,59.25 80.5,55.25 80.5,54.25 86.75,48 IC1.28
  Bottom 0.254: v76.25,59.25 74.75,59.25 73,61 73,67 67.5,72.5 40.5,72.5 39.56,73.44 R57.1
RX0  (via drill 0.2, 0.3)
  Top 0.254: v75.5,56.25 75.5,54 82.5,47 IC1.16 | v22.5,98.25 22.5,99.59 IRDA.P$3 | v53.5,98.5 53.5,108 53.35,108.15 SV3.6
  Bottom 0.254: v75.5,56.25 76.25,57 78.5,57 79,57.5 79,97.5 78,98.5 v53.5,98.5 22.75,98.5 v22.5,98.25
RXD  (via drill 0.2)
  Top 0.254: RS1.3 10.52,80.52 16.5,86.5 21.5,86.5 v23,85
  Bottom 0.254: D17.2 9.06,80.5 RS1.3 | v23,85 R62.2
SCL  (via drill 0.2, 0.3)
  Top 0.254: IC2.6 97.59,56.4 97.52,56.4 97.52,56.65 97.65,56.52 | IC2.6 97.64,53.63 v97.5,53.5 | IC1.38 89.75,53 v90.25,52.5 | R32.1 96.85,58.65 97.64,57.87 IC2.6
  Bottom 0.254: v97.5,53.5 | v90.25,52.5 91.25,53.5 v97.5,53.5 | v97.5,53.5
SDA  (via drill 0.2, 0.3)
  Top 0.254: 98.79,56.14 99.04,56.4 98.98,56.46 IC2.5 98.91,54.66 v98.75,54.5 | IC1.39 90.25,53.5 v91.25,54.5
  Top 0.406: IC2.5 98.91,63.09 98,64 96.92,64 R35.1
  Bottom 0.254: v98.75,54.5 | v91.25,54.5 v98.75,54.5 | v98.75,54.5
SEG0  (via drill 0.2, 0.3)
  Top 0.254: IC1.94 66,50 61.75,54.25 59.75,54.25 v57,57 | LCD1.1 24,63.5 30,69.5 v47.5,69.5
  Bottom 0.254: v47.5,69.5 47.5,62.5 53,57 v57,57
SEG1  (via drill 0.2, 0.3)
  Top 0.254: IC1.93 66.25,50.5 62,54.75 60.25,54.75 v58,57 | LCD1.2 26.5,63.5 31.5,68.5 v50,68.5
  Bottom 0.254: v50,68.5 50,62.5 54.5,58 57.5,58 58,57.5 v58,57
SEG2  (via drill 0.2, 0.3)
  Top 0.254: IC1.92 66.5,51 62.25,55.25 60.75,55.25 v59,57 | LCD1.3 29,63.5 33,67.5 v52.5,67.5
  Bottom 0.254: v52.5,67.5 52.5,62.5 56,59 58,59 59,58 v59,57
SEG3  (via drill 0.2, 0.3)
  Top 0.254: IC1.91 66.75,51.5 62.5,55.75 61.25,55.75 v60,57 | v55.12,66.5 34.5,66.5 31.5,63.5 LCD1.4
  Bottom 0.254: v55.12,66.5 55.12,62.5 57.62,60 58.5,60 60,58.5 v60,57
SEG4  (via drill 0.2, 0.3)
  Top 0.254: IC1.90 67,52 62.75,56.25 61.75,56.25 v61,57 | v57.62,65.5 36,65.5 34,63.5 LCD1.5
  Bottom 0.254: v57.62,65.5 57.62,62.5 61,59.12 v61,57
SEG5  (via drill 0.2, 0.3)
  Top 0.254: IC1.89 67.25,52.5 62.75,57 v62,57 | v60.25,64.5 37.5,64.5 36.5,63.5 LCD1.6
  Bottom 0.254: v60.25,64.5 60.25,61.5 62,59.75 v62,57
SEG6
  Top 0.254: IC1.88 67.5,53 62.5,58 44.58,58 39.08,63.5 LCD1.7
SEG7
  Top 0.254: IC1.87 67.75,53.5 62.75,58.5 46.62,58.5 41.62,63.5 LCD1.8
SEG8
  Top 0.254: IC1.86 68,54 63,59 48.66,59 44.16,63.5 LCD1.9
SEG9
  Top 0.254: IC1.85 68.25,54.5 63.25,59.5 50.7,59.5 46.7,63.5 LCD1.10
SEG10
  Top 0.254: IC1.84 68.5,55 63.5,60 52.74,60 49.24,63.5 LCD1.11
SEG11
  Top 0.254: IC1.83 68.75,55.5 63.75,60.5 54.78,60.5 51.78,63.5 LCD1.12
SEG12
  Top 0.254: IC1.82 69,56 64,61 56.82,61 54.32,63.5 LCD1.13
SEG13
  Top 0.254: IC1.81 69.25,56.5 64.25,61.5 58.86,61.5 56.86,63.5 LCD1.14
SEG14
  Top 0.254: IC1.80 69.5,57 64.5,62 60.9,62 59.4,63.5 LCD1.15
SEG15
  Top 0.254: IC1.79 69.75,57.5 64.75,62.5 62.94,62.5 61.94,63.5 LCD1.16
SEG16
  Top 0.254: IC1.78 69.98,58 69.98,58.02 64.5,63.5 LCD1.17
SEG17
  Top 0.254: IC1.77 70.25,58.5 66.52,62.23 LCD1.18
SEG18
  Top 0.254: IC1.76 70.5,59 69.06,60.44 LCD1.19
SEG19
  Top 0.254: IC1.73 76,62 75.5,62.5 73.1,62.5 72.1,63.5 LCD1.20
SEG20
  Top 0.254: IC1.72 76.5,62.25 75.25,63.5 LCD1.21
SEG21
  Top 0.254: IC1.71 77,63.18 LCD1.22
SEG22  (via drill 0.2)
  Top 0.254: IC1.70 77.5,59.5 78,59 v78.25,59
  Bottom 0.254: LCD1.23 76.68,87.32 77.5,86.5 77.5,64.5 78.5,63.5 78.5,59.25 v78.25,59
SEG23  (via drill 0.2)
  Top 0.254: IC1.69 78,63.5 | 78,63.5 | 78,63.5 78,63.75 76.75,65 v76.5,65
  Bottom 0.254: v76.5,65 76.5,86 74.14,88.36 LCD1.24
SEG24  (via drill 0.2)
  Top 0.254: IC1.68 78.5,64 76.5,66 v75.5,66
  Bottom 0.254: v75.5,66 75.5,79.75 61.78,93.47 LCD1.29
SEG25  (via drill 0.2)
  Top 0.254: IC1.67 79,64.25 76.25,67 v74.5,67
  Bottom 0.254: v74.5,67 74.5,80 62.25,92.25 60.25,92.25 59.03,93.47 LCD1.30
SEG26  (via drill 0.2)
  Top 0.254: IC1.66 79.5,64.5 76,68 v73.5,68
  Bottom 0.254: v73.5,68 73.5,80.25 62,91.75 58.25,91.75 56.53,93.47 LCD1.31
SEG27  (via drill 0.2)
  Top 0.254: IC1.65 80,64.75 75.75,69 v72.5,69
  Bottom 0.254: v72.5,69 72.5,80.5 61.75,91.25 56.25,91.25 54.03,93.47 LCD1.32
SEG28  (via drill 0.2)
  Top 0.254: IC1.64 80.5,65 75.5,70 v71.5,70
  Bottom 0.254: v71.5,70 71.5,80.75 61.5,90.75 54.25,90.75 51.53,93.47 LCD1.33
SEG29  (via drill 0.2)
  Top 0.254: IC1.63 81,65.25 75.25,71 v70.5,71
  Bottom 0.254: v70.5,71 70.5,81 61.25,90.25 52.25,90.25 49.03,93.47 LCD1.34
SEG30  (via drill 0.2)
  Top 0.254: IC1.62 81.5,65.5 75,72 v69.5,72
  Bottom 0.254: v69.5,72 69.5,81.25 61,89.75 50.25,89.75 46.53,93.47 LCD1.35
SEG31  (via drill 0.2)
  Top 0.254: IC1.61 82,65.75 74.75,73 v68.5,73
  Bottom 0.254: v68.5,73 68.5,81.5 60.75,89.25 48.25,89.25 44.03,93.47 LCD1.36
SEG32  (via drill 0.2)
  Top 0.254: IC1.60 82.5,66 74.5,74 v67.5,74
  Bottom 0.254: v67.5,74 67.5,81.75 60.5,88.75 46.25,88.75 41.53,93.47 LCD1.37
SEG33  (via drill 0.2)
  Top 0.254: IC1.59 83,66.25 74.25,75 v66.5,75
  Bottom 0.254: v66.5,75 66.5,82 60.25,88.25 44.25,88.25 39.03,93.47 LCD1.38
SEG34  (via drill 0.2)
  Top 0.254: IC1.58 83.5,66.5 74,76 v65.5,76 | LCD1.39 37.25,92.25 55.25,92.25 v60,87.5
  Bottom 0.254: v65.5,76 | v60,87.5 65.5,82 v65.5,76
SEG35  (via drill 0.2)
  Top 0.254: IC1.57 84,66.75 73.75,77 v64.5,77 | LCD1.40 33.53,93.47 35.25,91.75 54.25,91.75 v59.75,86.25
  Bottom 0.254: v64.5,77 | v59.75,86.25 64.5,81.5 v64.5,77
SEG36  (via drill 0.2)
  Top 0.254: IC1.56 84.5,67 73.5,78 v63.5,78 | LCD1.41 31.03,93.47 33.25,91.25 53.25,91.25 v59.5,85
  Bottom 0.254: v63.5,78 | v59.5,85 63.5,81 v63.5,78
SEG37  (via drill 0.2)
  Top 0.254: IC1.55 85,67.25 73.25,79 v62.5,79 | LCD1.42 28.53,93.47 31.25,90.75 52.25,90.75 v59.25,83.75
  Bottom 0.254: v62.5,79 | v59.25,83.75 62.5,80.5 v62.5,79
SEG38  (via drill 0.2)
  Top 0.254: 85.49,61.14 IC1.54 85.5,67.5 73,80 v61.5,80 | LCD1.43 26.03,93.47 29.25,90.25 51.25,90.25 v59,82.5
  Bottom 0.254: v61.5,80 | v59,82.5 v61.5,80
SEG39
  Top 0.254: 85.99,61.14 IC1.53 86,67.75 72.75,81 59,81 50.25,89.75 27.25,89.75 23.53,93.47 LCD1.44
TCK
  Top 0.254: JTAG.7 5.34,47.75 7.5,47.75 10.25,45 21.5,45 22.25,45.75 65.25,45.75 67,47.5 IC1.99
TDI
  Top 0.254: JTAG.3 5.42,52.75 7.5,52.75 8.5,51.75 8.5,48.25 10.75,46 21,46 21.75,46.75 64.75,46.75 66.5,48.5 IC1.97
TDO
  Top 0.254: JTAG.1 5.46,55.25 7.5,55.25 9,53.75 9,48.5 11,46.5 20.75,46.5 21.5,47.25 64.5,47.25 66.25,49 IC1.96
TEST  (via drill 0.3)
  Top 0.254: IC1.95 66,49.5 64.25,47.75 21.25,47.75 20.5,47 11.25,47 9.75,48.5 v9.75,49.75
  Bottom 0.254: v9.75,49.75 7.33,49.75 JTAG.8
TMS
  Top 0.254: JTAG.5 5.38,50.25 7.5,50.25 8,49.75 8,48 10.5,45.5 21.25,45.5 22,46.25 65,46.25 66.75,48 IC1.98
TX0  (via drill 0.2, 0.3)
  Top 0.254: v76.5,56.25 76.5,55.75 76.5,53.75 83,47.25 IC1.17 | v23.5,101 23.5,99.69 IRDA.P$2 | v52.5,99.5 v52.5,107.5
  Bottom 0.254: v76.5,56.25 78.5,56.25 79.5,57.25 79.5,59.25 79.5,62 79.5,62.5 79.5,96 | 79.5,96 79.5,95 | 79.5,96 79.5,98 78,99.5 v52.5,99.5 25,99.5 v23.5,101 | SV3.1 47,108.5 47.5,108 52,108 v52.5,107.5
TXD
  Bottom 0.254: RS1.2 9.27,78 R65.2 R66.1
V1
  Top 0.813: R16.2 R17.1
V1+
  Top 0.254: 72.25,42 72.5,42 75,44.5 IC1.1
  Top 0.406: C27.1 40.9,40.15 42.75,42 72.25,42
  Top 0.813: R19.2 C25.1 38.9,38.65 39.75,39.5 C27.1
V1-
  Top 0.254: IC1.2 75.5,44.25 72.25,41
  Top 0.406: C27.2 42.6,40.1 43.5,41 72.25,41
  Top 0.813: R20.1 C26.2 42.9,38.35 42.6,38.65 C27.2
VASYS
  Top 0.254: 79.5,43.48 IC1.10 | 79.5,43.48 C13.1 | 79.5,43.48 81.09,43.48 C11.2
VCORE
  Top 0.254: IC1.23 86,44 | IC1.23 | 86,44 | C14.2 87.15,42.85 86,44
VDSYS  (via drill 0.2)
  Top 0.254: IC1.74 75.5,61.75 75.25,62 73,62 72.75,61.75 72.75,61.27 C18.2 72.6,60.4 73,60 74,60 75.5,58.5 75.5,58 76,57.5 76.75,57.5 77.25,57 77.25,53.75 84.5,46.5 IC1.20 84.5,43.62 84.25,43.38 C9.2 84.9,42.73 85.56,42.06 C6.2 86.12,42.75 v85.38,43.5
  Bottom 0.254: v85.38,43.5 85.38,41.62 87.5,39.5 87.5,34.52 AUX3.1
VREF
  Top 0.254: IC1.7 78,43 77.5,42.5 C7.1 | C7.1
VSENSE  (via drill 0.3, 0.6)
  Top 0.254: v75.5,46.75 76.25,47.5 80.5,47.5 81.5,46.5 IC1.14
  Top 0.406: R31.2 R30.2 54.25,49.75 55,49 v62.25,49
  Bottom 0.254: v75.5,46.75 73.75,45 66.25,45 v62.25,49
VTEMP  (via drill 0.3, 0.6)
  Top 0.254: v74.75,47.5 75.25,48 80.75,48 82,46.75 IC1.15
  Top 0.406: R1.1 RTH.2 62.85,50.65 v63,50.5
  Bottom 0.254: v74.75,47.5 73.25,46 67.5,46 v63,50.5
XIN1
  Top 0.254: IC1.24 86.49,44.79 86.49,44.26 86.75,44 90.06,44 Q1.2
XOUT1
  Top 0.254: IC1.25 89.7,45.2 90,45.5 91.5,45.5 91.75,45.25 91.75,44.48 Q1.1

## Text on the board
tPlace: 120mA MAX
tNames: DVCC | DGND | DVCC | INTERNAL | MSP430F673x 1-Phase Energy Meter | Version 2.0 | EXTERNAL | DVCC | VCC_PL | VCC_EXT | RESET | GND | VCC_EXT | Max Thrun - June 2012 | 120/240 Vrms | Warning: | 60/50 Hz | 3VA | High Voltage
bNames: + | +
_tplace: R49 | SV1 | R53 | SV2 | R48 | DVCC | SV3 | DGND | R47 | R46 | C39 | R56 | R52 | C42 | R45 | C40 | R55 | R44 | R40 | R36 | R51 | R43 | C41 | R39 | R42 | R38 | JP5 | JP6 | RF2 | RF1 | R37 | OK2 | R54 | RS1 | IRDA | 1 | 1 | JP8 | R50 | REACT | OK1 | JP7 | 5 | 9 | 4 | R41 | 8 | 3 | ACT | 7 | 2 | 6 | LED2 | 1 | R5 | R4 | LCD1 | LED1 | R35 | JP1 | C37 | DVCC | R32 | 1 | INTERNAL | MSP430F673x 1-Phase Energy Meter | C18 | Version 2.4 | EXTERNAL | JP4 | DVCC | VCC_PL | IC1 | S1 | IC2 | VCC_EXT | R31 | R30 | R1 | RTH | R3 | C15 | C17 | RESET | C16 | C6 | R27 | C7 | C31 | R24 | C27 | C13 | C11 | C9 | C14 | R28 | R25 | Q1 | C30 | C25 | C26 | C19 | C23 | C21 | C24 | C2 | C4 | R26 | R29 | C1 | C3 | U1 | R19 | R20 | R12 | C20 | R14 | C22 | JTAG | * | C35 | R18 | R17 | R9 | R13 | R10 | R15 | D13 | R23 | R11 | R16 | R7 | R8 | C32 | D11 | D12 | JP2 | C33 | C34 | AUX1 | AUX2 | AUX3 | L3 | L4 | L5 | L6 | R21 | D9 | D10 | JP3 | GND | C28 | R34 | VCC_EXT | D2 | D4 | D6 | D8 | C38 | D1 | D3 | D5 | D7 | S3 | R22 | R6 | R33 | L1 | L2 | 120mA MAX | S2 | C36 | LINE | NEUTRAL | 120/240 Vrms | Warning: | CUR1+ | CUR1- | CUR2+ | CUR2- | 60/50 Hz | 3VA | High Voltage
_bplace: D15 | + | C44 | R62 | D16 | C45 | + | U2 | D17 | C43 | D14 | R58 | R59 | T1 | R61 | R65 | R60 | R66 | T2 | R64 | R63 | R57 | U3 | R2 | C8 | C10 | C29 | C5 | C12 | L7 | ELLCTV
